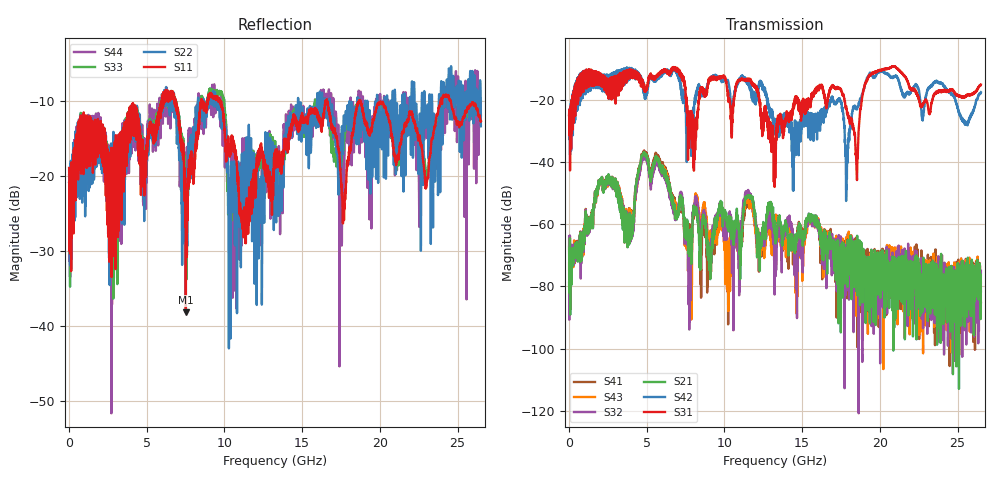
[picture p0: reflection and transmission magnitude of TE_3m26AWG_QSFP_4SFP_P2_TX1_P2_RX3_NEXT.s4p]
!Agilent Technologies,N5222A,MY51421691,A.10.00.00
!Agilent N5222A: A.10.00.00
!Date: Friday, January 30, 2015 12:35:45
!Correction: S11(Full 4 Port(1,2,3,4))
!S12(Full 4 Port(1,2,3,4))
!S13(Full 4 Port(1,2,3,4))
!S14(Full 4 Port(1,2,3,4))
!S21(Full 4 Port(1,2,3,4))
!S22(Full 4 Port(1,2,3,4))
!S23(Full 4 Port(1,2,3,4))
!S24(Full 4 Port(1,2,3,4))
!S31(Full 4 Port(1,2,3,4))
!S32(Full 4 Port(1,2,3,4))
!S33(Full 4 Port(1,2,3,4))
!S34(Full 4 Port(1,2,3,4))
!S41(Full 4 Port(1,2,3,4))
!S42(Full 4 Port(1,2,3,4))
!S43(Full 4 Port(1,2,3,4))
!S44(Full 4 Port(1,2,3,4))
!S4P File: Measurements: <S11,S12,S13,S14>,
!<S21,S22,S23,S24>,
!<S31,S32,S33,S34>,
!<S41,S42,S43,S44>:
# Hz S  dB  R 50.0
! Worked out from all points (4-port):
!   2650 points, 10 MHz to 26.5 GHz, reference 50 ohm
!   strongest paths, dB at 10 MHz, 6.63 GHz, 13.26 GHz, 19.88 GHz, 26.5 GHz:
!     S31: -24.9, -10.3, -36.2, -10.8, -15.2
!     S42: -25.0, -10.8, -28.8, -11.2, -17.6
!     S21: -78.8, -53.1, -62.5, -82.6, -81.7
!     S32: -63.8, -54.3, -67.2, -89.0, -75.0
!     S43: -72.7, -53.6, -58.8, -83.3, -78.9
!     S41: -67.3, -52.1, -57.5, -75.6, -85.1
!   lowest |S11| = -38.2 dB at 7.52 GHz (marker M1), VSWR 1.02, Z = 51.2 + j0.159 ohm
!   |S11| at or under -10 dB: start of sweep to 5.957 GHz; 9.721 GHz to 16.5 GHz (6.778 GHz wide, 51.7 % of centre); 18.76 GHz to 23.91 GHz (5.149 GHz wide, 24.1 % of centre)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
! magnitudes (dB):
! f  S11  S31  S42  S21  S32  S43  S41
! 10 MHz  -18.9  -24.9  -25.0  -78.8  -63.8  -72.7  -67.3
! 4.79 GHz  -17.2  -16.0  -14.4  -37.3  -38.8  -38.2  -36.7
! 7.52 GHz  -38.2  -19.8  -22.1  -60.7  -60.1  -59.8  -60.5
! 17.33 GHz  -16.5  -16.4  -20.2  -70.2  -70.0  -68.4  -73.1
! 18.49 GHz  -11.0  -41.8  -23.0  -68.6  -74.3  -76.3  -65.8
! 19.59 GHz  -12.4  -11.4  -12.7  -91.4  -71.6  -78.0  -69.3
! 26.5 GHz  -12.7  -15.2  -17.6  -81.7  -75.0  -78.9  -85.1
